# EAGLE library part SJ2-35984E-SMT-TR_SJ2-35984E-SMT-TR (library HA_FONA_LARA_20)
4 conductors, 3.5mm, SMT Audio Jack w/ 3 Switch
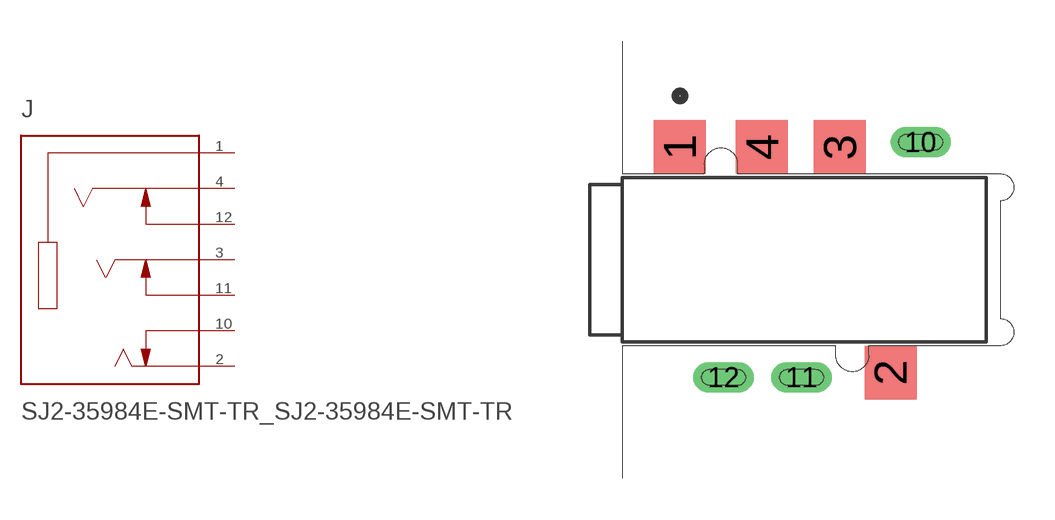
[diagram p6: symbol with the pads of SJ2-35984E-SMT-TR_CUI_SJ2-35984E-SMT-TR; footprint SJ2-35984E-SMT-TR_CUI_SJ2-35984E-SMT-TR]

Designator prefix J

## SJ2-35984E-SMT-TR_SJ2-35984E-SMT-TR (MANUFACTURER: CUI; STANDARD: Manufacturer recommendation)  [SJ2-35984E-SMT-TR_CUI_SJ2-35984E-SMT-TR]
1  SLEEVE  pas
2  TIP  pas
3  RING1  pas
4  RING2  pas
10  TIP_SWITCH  pas
11  RING1_SWITCH  pas
12  RING2_SWITCH  pas

## Footprint SJ2-35984E-SMT-TR_CUI_SJ2-35984E-SMT-TR (pad centres in mm)
smd 1.9 x 1.95: 1 -4.55,4.125; 2 3.15,-4.125; 3 1.3,4.125; 4 -1.55,4.125
drill 0.6 long: 10 4.25,4.3; 11 -0.1,-4.3; 12 -2.95,-4.3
